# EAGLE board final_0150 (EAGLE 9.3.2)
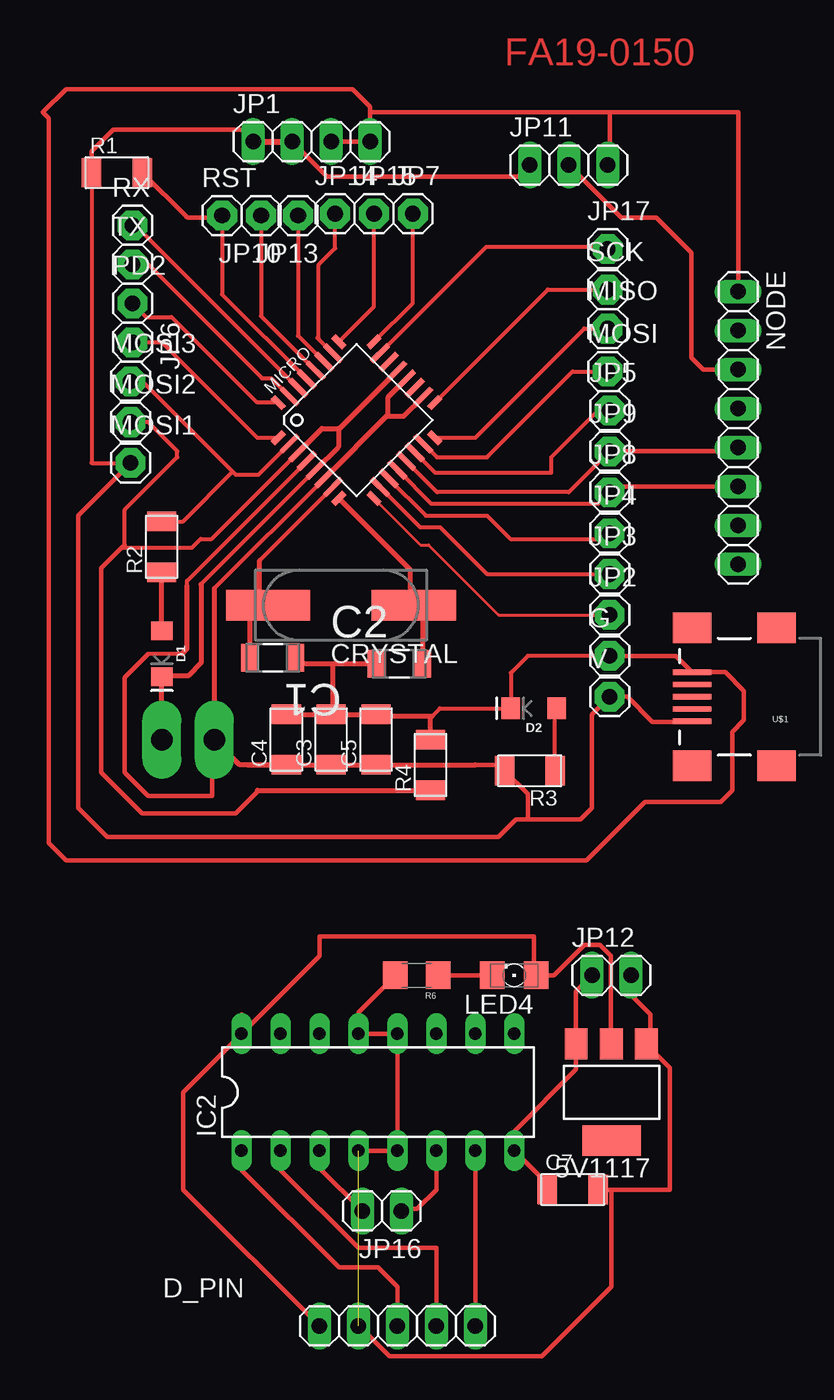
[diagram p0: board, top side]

No outline drawn. Coordinates in mm, seen from the top.
Copper layers (1*16): Top 0.035mm / dielectric 1.5mm / Bottom 0.035mm
Design rules "default": minimum track width 6mil, minimum drill 0.35mm, track to track 6mil, track to pad 6mil, pad to pad 6mil, via to via 6mil, smd to smd 6mil, copper to edge 40mil, drill to drill 6mil, minimum pad ring 10mil, minimum via ring 8mil, stop-mask expansion 4mil, vias tented up to drill 0mil, thermal gap 10mil

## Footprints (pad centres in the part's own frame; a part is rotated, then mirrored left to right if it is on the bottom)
SOT223 = smd 1.499 x 2.007: 1 -2.261,-3.15; 2 0.025,-3.15; 3 2.311,-3.15 | smd 3.81 x 2.007: 4 0,3.15
CAPC3216X178N = smd 1.118 x 1.803: 1 -1.499,0; 2 1.499,0
C1206FAB = smd 1.27 x 1.905: 1 -1.651,0; 2 1.651,0
CSM-7X-DU = smd 5.5 x 2: 1 -4.75,0; 2 4.75,0
LED-1206 = smd 1.2 x 1.4: A -1.5,0; C 1.5,0
1X05 = drill 1.016 long: 1 -5.08,0; 2 -2.54,0; 3 0,0; 4 2.54,0; 5 5.08,0
1X01 = drill 1.016 pad 1.93 octagon: 1 0,0
1X1-BIGPOGO = drill 1.4 pad 2.54 long: P$1 0,0
DIL16 = drill 0.813 long: 1 -8.89,-3.81; 2 -6.35,-3.81; 3 -3.81,-3.81; 4 -1.27,-3.81; 5 1.27,-3.81; 6 3.81,-3.81; 7 6.35,-3.81; 8 8.89,-3.81; 9 8.89,3.81; 10 6.35,3.81; 11 3.81,3.81; 12 1.27,3.81; 13 -1.27,3.81; 14 -3.81,3.81; 15 -6.35,3.81; 16 -8.89,3.81
1X04 = drill 1.016 long: 1 -3.81,0; 2 -1.27,0; 3 1.27,0; 4 3.81,0
1X03 = drill 1.016 long: 1 -2.54,0; 2 0,0; 3 2.54,0
1X02 = drill 1.016 long: 1 -1.27,0; 2 1.27,0
1206 = smd 1.6 x 1.803: A -1.422,0; C 1.422,0
TQFP32-08 = smd 1.016 x 0.406: 1 -4.42,2.8; 8 -4.42,-2.8; 17 4.42,-2.8; 24 4.42,2.8 | smd 1.524 x 0.356: 2 -4.166,2; 3 -4.166,1.2; 4 -4.166,0.4; 5 -4.166,-0.4; 6 -4.166,-1.2; 7 -4.166,-2; 18 4.166,-2; 19 4.166,-1.2; 20 4.166,-0.4; 21 4.166,0.4; 22 4.166,1.2; 23 4.166,2 | smd 0.406 x 1.016: 9 -2.8,-4.42; 16 2.8,-4.42; 25 2.8,4.42; 32 -2.8,4.42 | smd 0.356 x 1.524: 10 -2,-4.166; 11 -1.2,-4.166; 12 -0.4,-4.166; 13 0.4,-4.166; 14 1.2,-4.166; 15 2,-4.166; 26 2,4.166; 27 1.2,4.166; 28 0.4,4.166; 29 -0.4,4.166; 30 -1.2,4.166; 31 -2,4.166
1X08 = drill 1.016 long: 1 -8.89,0; 2 -6.35,0; 3 -3.81,0; 4 -1.27,0; 5 1.27,0; 6 3.81,0; 7 6.35,0; 8 8.89,0
R1206FAB = smd 1.27 x 1.905: 1 -1.651,0; 2 1.651,0
1206' = smd 1.6 x 1.8: 1 -1.4,0; 2 1.4,0
USB_MINIB = smd 2.5 x 0.35: D+ 3.77,0; D- 3.77,0.8; GND 3.77,-1.6; ID 3.77,-0.8; VBUS 3.77,1.6 | smd 2.5 x 2: SHIELD@1 -1.73,-4.5; SHIELD@2 -1.73,4.5; SHIELD@3 3.77,4.5; SHIELD@4 3.77,-4.5

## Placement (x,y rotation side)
5V1117  REG1117  [SOT223]  104.14,-31.75 180 top
C1  22pF  [CAPC3216X178N]  82.04,-3.43 180 top
C2  22pF  [CAPC3216X178N]  90.3,-3.81 0 top
C3  10uF  [C1206FAB]  85.85,-8.76 90 top
C4  1uF  [C1206FAB]  82.93,-8.76 90 top
C5  100nF  [C1206FAB]  88.77,-8.76 90 top
C7  10uF  [C1206FAB]  101.6,-38.1 0 top
CRYSTAL  16Mhz  [CSM-7X-DU]  86.49,0 180 top
D1  RED  [LED-1206]  74.8,-3.17 270 top
D2  Green  [LED-1206]  99.06,-6.73 180 top
D_PIN  [1X05]  90.17,-46.99 0 top
G  [1X01]  104.01,-3.3 0 top
GND  [1X1-BIGPOGO]  74.8,-8.76 90 top
IC2  L293D  [DIL16]  88.9,-31.75 0 top
JP1  [1X04]  84.58,30.23 0 top
JP2  [1X01]  104.01,-0.64 0 top
JP3  [1X01]  104.01,2.03 0 top
JP4  [1X01]  104.01,4.7 0 top
JP5  [1X01]  104.01,12.7 0 top
JP6  [1X01]  72.9,17.14 269.6 top
JP7  [1X01]  91.19,25.53 0 top
JP8  [1X01]  104.01,7.37 0 top
JP9  [1X01]  104.01,10.03 0 top
JP10  [1X01]  81.28,25.4 180 top
JP11  [1X03]  101.35,28.7 0 top
JP12  [1X02]  104.14,-24.13 0 top
JP13  [1X01]  83.69,25.4 180 top
JP14  [1X01]  86.11,25.53 0 top
JP15  [1X01]  88.65,25.53 0 top
JP16  [1X02]  89.15,-39.5 180 top
JP17  [1X01]  103.89,23.24 0 top
LED4  [1206]  97.79,-24.13 180 top
MICRO  ATMEGA328P-AU  [TQFP32-08]  87.5,12.06 45 top
MISO  [1X01]  103.89,18.03 0 top
MOSI  [1X01]  103.89,15.24 0 top
MOSI1  [1X01]  72.77,9.27 0 top
MOSI2  [1X01]  72.77,11.94 0 top
MOSI3  [1X01]  72.77,14.61 0 top
NODE  [1X08]  112.39,11.56 270 top
PD2  [1X01]  72.9,19.68 0 top
R1  10k  [R1206FAB]  71.88,28.19 0 top
R2  1k  [R1206FAB]  74.8,3.81 90 top
R3  499  [R1206FAB]  98.81,-10.79 180 top
R4  0  [R1206FAB]  92.33,-10.41 90 top
R6  499  [1206']  91.44,-24.13 180 top
RST  [1X01]  78.74,25.4 0 top
RX  [1X01]  72.9,24.77 0 top
SCK  [1X01]  103.89,20.57 0 top
TX  [1X01]  72.9,22.23 0 top
U$1  USB_MINIB  [USB_MINIB]  113.16,-5.97 180 top
V  [1X01]  104.01,-5.97 0 top
VCC  [1X1-BIGPOGO]  78.23,-8.76 90 top

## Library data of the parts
5V1117 = burr-brown; MPN: REG1117; OC_FARNELL: 1097566; OC_NEWARK: 14P6981
C1 C2 = AVX_By_element14_Batch_1; MPN: 0612ZC225MAT2A; OC_FARNELL: -; OC_NEWARK: 12N3209; SUPPLIER: AVX; TOLERANCE: ±20%; VOLTAGERATING: 10V
C3-C5 R1-R4 U$1 = fab
C7 = fab (1)
CRYSTAL = 01_FAB_Hello; OC_FARNELL: unknown; OC_NEWARK: unknown
D1 D2 = SparkFun-LED; PROD_ID: DIO-09912
D_PIN JP1 JP11 JP12 JP16 NODE = pinhead
G GND JP2-JP10 JP13-JP15 JP17 MISO MOSI MOSI1-MOSI3 PD2 RST RX SCK TX V VCC = adafruit
IC2 = st-microelectronics; MPN: L293D; OC_FARNELL: 9589619; OC_NEWARK: 56P8249
LED4 = led
MICRO = atmega8
R6 = 01_SparkFun

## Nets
1: JP2.1 MICRO.9
2: JP3.1 MICRO.10
3: JP4.1 MICRO.11
4: JP8.1 MICRO.12 NODE.6
5: JP9.1 MICRO.13 NODE.5
12V: 5V1117.3 C7.1 IC2.8 JP12.1
ADC6: MICRO.19
ADC7: MICRO.22
GND: C1.1 C2.1 C3.2 C4.2 C5.2 D1.C D2.C G.1 GND.P$1 JP1.3 JP1.4 JP11.3 MICRO.3 MICRO.5 MICRO.21 MOSI2.1 NODE.1 R4.1 R4.2 U$1.GND
GND1: 5V1117.1 C7.2 D_PIN.2 IC2.4 IC2.5 IC2.12 IC2.13 JP12.2 R6.2
LED: MICRO.2 MOSI3.1 R2.2
M5: D_PIN.5 IC2.7
M6: D_PIN.4 IC2.2
M7: IC2.15
M8: IC2.10
MISO: MICRO.16 MISO.1
MOSI: MICRO.15 MOSI.1
N5: IC2.6 JP16.1
N6: IC2.3 JP16.2
N7: IC2.14
N8: IC2.11
N$1: D2.A R3.1
N$2: C1.2 CRYSTAL.2 MICRO.7
N$3: MICRO.29 R1.2 RST.1
N$4: LED4.C R6.1
N$5: NODE.2
N$7: NODE.4
N$8: JP11.2 NODE.3
N$9: C2.2 CRYSTAL.1 MICRO.8
N$11: NODE.7
N$12: NODE.8
N$25: D1.A R2.1
PB2: JP5.1 MICRO.14
PC0: JP17.1 MICRO.23
PC1: JP7.1 MICRO.24
PC2: JP15.1 MICRO.25
PC3: JP14.1 MICRO.26
PC4: JP13.1 MICRO.27
PC5: JP10.1 MICRO.28
PD2: MICRO.32 PD2.1
PD3: JP6.1 MICRO.1
PWM2: D_PIN.3 IC2.1
RX: MICRO.30 RX.1
SCK: MICRO.17 SCK.1
TX: MICRO.31 TX.1
VCC: C3.1 C4.1 C5.1 JP1.1 JP1.2 JP11.1 MICRO.4 MICRO.6 MICRO.18 MICRO.20 MOSI1.1 R1.1 R3.2 U$1.VBUS V.1 VCC.P$1
VCC1: 5V1117.2 D_PIN.1 IC2.16 LED4.A

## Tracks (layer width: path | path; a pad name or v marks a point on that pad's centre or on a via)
1
  Top 0.203: MICRO.9 91.67,3.94 92.2,3.94 96.77,-0.64 JP2.1
2
  Top 0.254: MICRO.10 91.66,5.08 92.96,5.08 96.01,2.03 JP3.1 104.78,2.03
3
  Top 0.254: JP4.1 103.82,4.51 103.63,4.32 97.54,4.32 96.01,5.84 92.03,5.84 MICRO.11
4
  Top 0.254: 103.63,6.6 103.63,6.99 JP8.1 103.25,6.6 92.4,6.6 MICRO.12
  Top 0.3: NODE.6 104.39,7.75 JP8.1
5
  Top 0.254: JP9.1 101.35,7.37 92.77,7.37 MICRO.13
  Top 0.3: JP9.1 112.14,10.03 NODE.5
12V
  Top 0.3: C7.1 99.95,-37.72 IC2.8 97.79,-34.29 101.83,-30.25 5V1117.3 101.83,-25.17 JP12.1
GND
  Top 0.254: G.1 98.68,-3.3 97.56,-4.42 D2.C 92.94,-6.73 92.33,-7.34 | 72.39,3.94 72.39,6.22 75.82,9.65 75.82,10.03 73.91,11.94 MOSI2.1 | 72.2,3.75 76.77,3.75 77.34,4.32 78.06,4.32 83.99,10.25 | MICRO.5 77.37,1.37
  Top 0.3: JP1.4 88.39,32.51 87.25,33.66 68.58,33.66 67.06,32.13 67.44,31.75 67.44,-15.49 68.58,-16.64 102.49,-16.64 106.3,-12.83 111.25,-12.83 112.01,-12.06 112.01,-8.26 112.78,-7.49 112.78,-5.59 111.56,-4.37 U$1.GND 108.32,-3.3 G.1 | JP1.4 JP1.3 | NODE.1 112.39,32.13 104.01,32.13 | 104.01,32.13 88.39,32.13 JP1.4 | 104.01,32.13 104.01,28.7 | 104.39,28.32 104.01,28.7 | 104.01,28.7 JP11.3
  Top 0.305: 72.39,3.94 72.2,3.75 70.87,2.41 70.87,-10.92 73.53,-13.59 79.63,-13.59 81.03,-12.19 81.03,-12.06
  Top 0.33: 74.57,-4.67 D1.C | D1.C 74.42,-5.06 | MICRO.3 83.99,10.25 85.26,11.52 86.32,11.52 | C1.1 83.92,-3.81 85.98,-3.81 | 85.98,-3.81 C2.1 | GND.P$1 D1.C | D1.C 74.91,-4.57 76.58,-4.57 77.37,-3.78 77.37,1.37 | 81.03,-12.06 R4.1 | C3.2 85.72,-6.99 | C4.2 C3.2 | C3.2 C5.2 88.39,-7.24 92.43,-7.24 92.33,-7.34 R4.2 | C3.2 85.98,-6.99 85.98,-3.81 | 86.32,11.52 86.32,10.32 MICRO.5 | MICRO.21 86.39,11.52 86.32,11.52
GND1  (1 unrouted)
  Top 0.3: R6.2 87.63,-26.54 IC2.13 IC2.12 IC2.5 IC2.4 | C7.2 104.14,-38.1 107.95,-38.1 107.95,-30.15 106.68,-28.88 | 106.68,-28.88 5V1117.1 | JP12.2 105.41,-25.4 106.68,-26.67 106.68,-28.88
  Top 0.305: D_PIN.2 87.67,-46.99 89.66,-48.98 99.61,-48.98 104.14,-44.45 104.14,-38.1
LED
  Top 0.254: MOSI3.1 73.53,14.61 79.44,8.7 | 79.44,8.7 79.63,8.51 81.12,8.51 MICRO.2 | R2.2 76.2,5.46 79.44,8.7
M5
  Top 0.305: IC2.7 D_PIN.5
M6
  Top 0.305: D_PIN.4 92.71,-41.91 87.63,-41.91 82.55,-36.83 IC2.2
MISO
  Top 0.254: MISO.1 102.36,18.03 95.25,10.92 MICRO.16
MOSI
  Top 0.254: MOSI.1 101.6,15.24 96.01,9.65 92.74,9.65 MICRO.15
N5
  Top 0.305: IC2.6 92.71,-38.1 91.44,-39.37 90.55,-39.37 JP16.1
N6
  Top 0.305: IC2.3 85.09,-36.7 JP16.2
N$1
  Top 0.254: R3.1 100.46,-6.83 D2.A
N$2
  Top 0.254: 81.19,2.93 MICRO.7
  Top 0.33: CRYSTAL.2 81.19,-0.43 | 81.19,-0.43 80.52,-0.96 80.52,-3.94 80.54,-3.91 C1.2 | 81.19,-0.43 81.19,2.93
N$3
  Top 0.254: MICRO.29 78.74,20.26 RST.1
  Top 0.305: RST.1 78.74,25.27 76.56,25.27 arc-45 76.38,25.35 R1.2
N$4
  Top 0.3: R6.1 LED4.C 96.52,-24.13
N$8
  Top 0.3: JP11.2 104.78,25.27 107.06,25.27 109.35,22.99 109.35,16.13 110.11,15.37 NODE.3
N$9
  Top 0.33: MICRO.8 90.98,2.33 90.98,0.25 CRYSTAL.1 91.8,-0.81 C2.2
N$25
  Top 0.33: D1.A R2.1
PB2
  Top 0.254: JP5.1 103.25,12.7 100.2,9.65 100.2,8.64 92.63,8.64 MICRO.14
PC0
  Top 0.254: 89.07,16.43 MICRO.23 95.98,23.37 103.76,23.37 JP17.1
PC1
  Top 0.254: JP7.1 91.19,19.71 MICRO.24
PC2
  Top 0.254: JP15.1 88.65,19.46 MICRO.25
PC3
  Top 0.254: MICRO.26 85.04,17.35 | 85.04,17.35 84.96,17.43 | 85.04,17.35 85.04,22.2 86.11,23.26 JP14.1
PC4
  Top 0.254: MICRO.27 83.72,17.55 | 83.72,17.55 83.69,17.57 | 83.72,17.55 83.72,25.38 JP13.1
PC5
  Top 0.254: MICRO.28 81.28,18.85 JP10.1
PD2
  Top 0.254: PD2.1 73.79,18.8 75.44,18.8 81.02,13.21 MICRO.32
PD3
  Top 0.254: JP6.1 74.8,17.14 81.03,10.92 MICRO.1
PWM2
  Top 0.305: D_PIN.3 90.17,-44.45 88.9,-43.18 86.36,-43.18 80.01,-36.83 IC2.1
RX
  Top 0.254: MICRO.30 73.15,24.72 73.15,24.77
  Top 0.305: RX.1 73.15,24.77 73.28,24.77
SCK
  Top 0.254: MICRO.17 99.97,20.57 SCK.1
TX
  Top 0.254: TX.1 73.91,22.23 81.34,14.8 81.94,14.8 MICRO.31
VCC
  Top 0.254: R1.1 70.23,9.27 MOSI1.1 | 76.11,-3.17 73.91,-3.17 | MICRO.6 78.23,1.1 | 76.45,1.27 76.45,1.58 MICRO.4
  Top 0.3: JP1.2 85.6,27.94 98.04,27.94 JP11.1 | V.1 105.16,-5.97 106.81,-7.62 109.34,-7.62 U$1.VBUS
  Top 0.305: R1.1 70.23,29.59 71.63,30.99 80.01,30.99 JP1.1 | 73.91,-3.17 72.39,-4.7 72.39,-10.92 73.91,-12.45 78.11,-12.45 78.11,-8.38 78.23,-8.26 | MOSI1.1 69.34,5.84 69.34,-13.21 71.25,-15.11 96.77,-15.11 97.92,-13.97 98.68,-13.97 | 95.25,-10.41 96.77,-10.41 R3.2 98.68,-12.32 98.68,-13.97 | 98.68,-13.97 102.11,-13.97 102.87,-13.21 102.87,-7.11 V.1
  Top 0.33: C4.1 C3.1 C5.1 95.25,-10.41 | 80.39,-10.41 C4.1 | 76.11,-3.17 76.45,-2.83 76.45,1.27 | C4.1 79.88,-10.41 VCC.P$1 | MICRO.20 89.53,13.53 89.53,12.4 | 89.53,12.4 89.53,12.32 90.58,12.32 MICRO.18 | MICRO.6 89.53,12.4 | 78.23,1.1 78.23,-8.26 VCC.P$1 | VCC.P$1 78.11,-8.89
  Top 0.406: JP1.1 JP1.2
VCC1
  Top 0.3: 5V1117.2 104.1,-28.58 | 104.1,-25.4 104.1,-22.86 103.38,-22.14 102.36,-22.14 100.37,-24.13 LED4.A
  Top 0.305: 104.1,-28.58 104.1,-25.4 | 80.01,-26.67 IC2.16 | IC2.16 85.09,-22.86 85.09,-21.59 99.06,-21.59 99.06,-23.98 LED4.A | IC2.16 76.2,-31.75 76.2,-38.1 D_PIN.1

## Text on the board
Top: FA19-0150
